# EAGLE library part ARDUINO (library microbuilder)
Arduino Diecimila/Duemilanove Make a shield with ease, this package has all the named pins as well as the two mounting drill holes and an outline of the USB and DC power connector. The outline is on the DIMENSION layer, so if your board house uses it they will cut the outline to match. http://www.ladyada.net/library/pcb/eaglelibrary.html
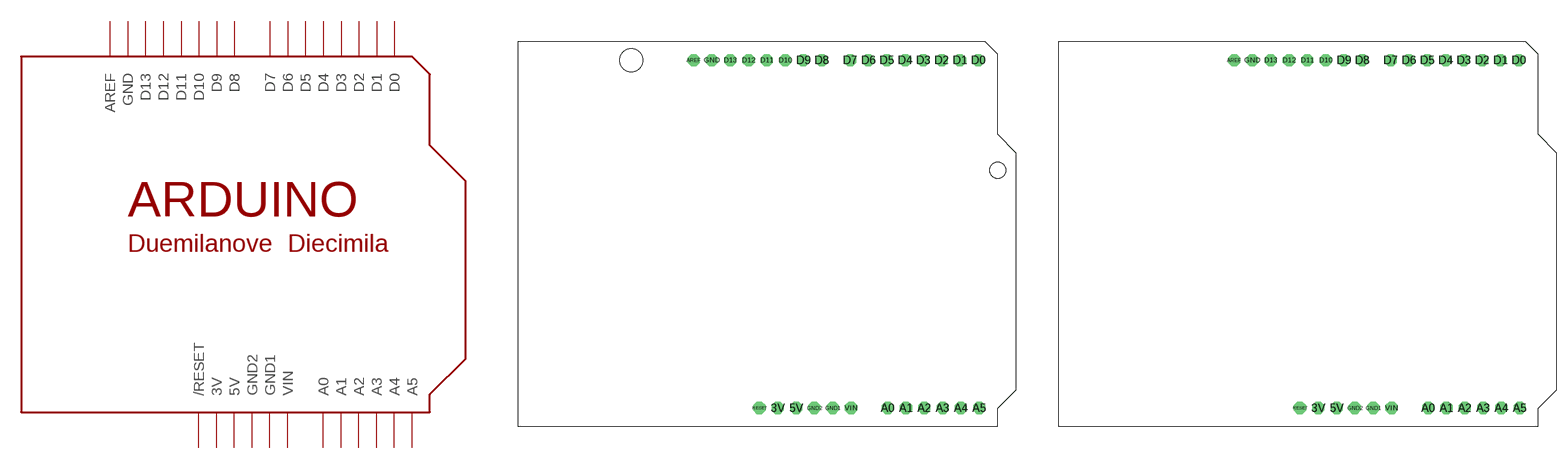
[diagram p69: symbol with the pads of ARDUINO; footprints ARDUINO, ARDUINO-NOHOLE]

Designator prefix -

## ARDUINODUEMILANOVE  [ARDUINO]
3V  3V  pwr
5V  5V  pwr
A0  A0
A1  A1
A2  A2
A3  A3
A4  A4
A5  A5
AREF  AREF
D0  D0
D1  D1
D2  D2
D3  D3
D4  D4
D5  D5
D6  D6
D7  D7
D8  D8
D9  D9
D10  D10
D11  D11
D12  D12
D13  D13
GND  GND  pwr
GND1  GND1  pwr
GND2  GND2  pwr
RESET  /RESET
VIN  VIN  pwr

## ARDUINODUEMILANOVE-NOHOLES  [ARDUINO-NOHOLE]
Pads as for ARDUINO

## ARDUINODUEMILANOVE-NODIM  [ARDUINO-NODIM]
Pads as for ARDUINO

## Footprint ARDUINO (pad centres in mm)
Arduino Diecimila/Duemilanove Make a shield with ease, this package has all the named pins as well as the two mounting drill holes and an outline of the USB and DC power connector. The outline is on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
drill 1 pad 1.676 octagon: 3V 36.068,2.54; 5V 38.608,2.54; A0 51.308,2.54; A1 53.848,2.54; A2 56.388,2.54; A3 58.928,2.54; A4 61.468,2.54; A5 64.008,2.54; AREF 24.384,50.8; D0 63.881,50.8; D1 61.341,50.8; D2 58.801,50.8; D3 56.261,50.8; D4 53.721,50.8; D5 51.181,50.8; D6 48.641,50.8; D7 46.101,50.8; D8 42.164,50.8; D9 39.624,50.8; D10 37.084,50.8; D11 34.544,50.8; D12 32.004,50.8; D13 29.464,50.8; GND 26.924,50.8; GND1 43.688,2.54; GND2 41.148,2.54; RESET 33.528,2.54; VIN 46.228,2.54
hole 3.2 at 15.758,50.754
hole 2.2 at 66.558,35.514

## Footprint ARDUINO-NOHOLE (pad centres in mm)
drill 1 pad 1.676 octagon: 3V 36.068,2.54; 5V 38.608,2.54; A0 51.308,2.54; A1 53.848,2.54; A2 56.388,2.54; A3 58.928,2.54; A4 61.468,2.54; A5 64.008,2.54; AREF 24.384,50.8; D0 63.881,50.8; D1 61.341,50.8; D2 58.801,50.8; D3 56.261,50.8; D4 53.721,50.8; D5 51.181,50.8; D6 48.641,50.8; D7 46.101,50.8; D8 42.164,50.8; D9 39.624,50.8; D10 37.084,50.8; D11 34.544,50.8; D12 32.004,50.8; D13 29.464,50.8; GND 26.924,50.8; GND1 43.688,2.54; GND2 41.148,2.54; RESET 33.528,2.54; VIN 46.228,2.54

## Footprint ARDUINO-NODIM (pad centres in mm)
drill 1 pad 1.676 octagon: 3V 36.068,2.54; 5V 38.608,2.54; A0 51.308,2.54; A1 53.848,2.54; A2 56.388,2.54; A3 58.928,2.54; A4 61.468,2.54; A5 64.008,2.54; AREF 24.384,50.8; D0 63.881,50.8; D1 61.341,50.8; D2 58.801,50.8; D3 56.261,50.8; D4 53.721,50.8; D5 51.181,50.8; D6 48.641,50.8; D7 46.101,50.8; D8 42.164,50.8; D9 39.624,50.8; D10 37.084,50.8; D11 34.544,50.8; D12 32.004,50.8; D13 29.464,50.8; GND 26.924,50.8; GND1 43.688,2.54; GND2 41.148,2.54; RESET 33.528,2.54; VIN 46.228,2.54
